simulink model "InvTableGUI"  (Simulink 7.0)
settings: Solver=FixedStepDiscrete  StartTime=0.0  StopTime=inf  FixedStep=samplePeriod  RelTol=1e-3
PreLoadFcn:
  | initialize
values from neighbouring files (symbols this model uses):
  forceCanon = 0.00444822    [initialize.m]    (also in TableInit.m = 1)
  iactParams = [	actParams    [initialize.m]
  inertia = inertia + inertiaP2Q([0 0 0], massA(i), cgA(:,i)-cg,  									inertiaCanon, massCanon)    [initialize.m]    (also in TableInit.m = [Ixx 0 0; 0 Iyy 0; 0 0 Izz])
  inertiaMask = zeros(3, 1)    [initialize.m]
  initDispl = zeros(6, 1)    [initialize.m]
  lengthCanon = 25.4    [initialize.m]    (also in TableInit.m)
  mass = ones(3, 1) * (sum(massA) + massT + massS)    [initialize.m]    (also in TableInit.m = 17300)
  massMask = zeros(3, 1)    [initialize.m]
  pitch = drot(2) * canon    [animation.m]    (also in positT2A.m = tbl(5))
  returnPress = 50    [initialize.m]    (also in TableInit.m)
  roll = drot(1) * canon    [animation.m]    (also in positT2A.m = tbl(4))
  rtg = cg    [initialize.m]    (also in TableInit.m = [0 0 cg])
  samplePeriod = controlPeriod/upsampleFactor    (= 0.00048828125)    [initialize.m]    (also in viewer.m = eval(getHeaderValue(header, 'DELTA_T')); TableInit.m = 0.0009765625)
  staticForce = forceT2A(ftbl, dtbl0, dof, rh, rb, rl, canon, atype)    [initialize.m]
undefined symbols (not defined in the file or in its folder): animation, atype, DiscIntNeverNeededParam, friction, yieldDispl
libraries: LibTransforms x15, LibDynamics x12, simulink x1

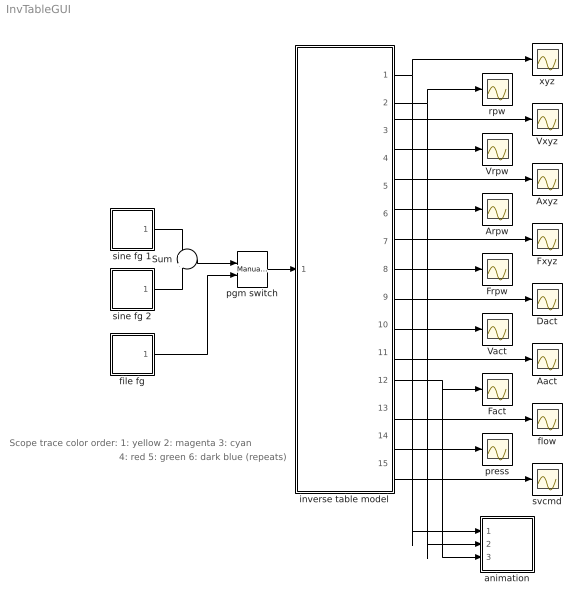
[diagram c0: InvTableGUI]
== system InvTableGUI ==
  note: Scope trace color order: 1: yellow 2: magenta 3: cyan
  note: 4: red 5: green 6: dark blue (repeats)
  Aact : Scope
  Arpw : Scope
  Axyz : Scope
  Dact : Scope
  Fact : Scope
  Frpw : Scope
  Fxyz : Scope
  Sum : Sum  Inputs=+|+  OutDataType=sfix(16)  OutScaling=2^0
  Vact : Scope
  Vrpw : Scope
  Vxyz : Scope
  animation : Subsystem  mask{azim=-37.5, elev=35, params=animation, decim=ceil((1/samplePeriod)/32), samplePeriod=samplePeriod}
      mask prompts: azim "View azimuth (degrees)"; elev "View elevation (degrees)"; params "Parameters"; decim "Decimation factor"; samplePeriod "Sample period (sec)"
  file fg : Subsystem
  flow : Scope
  inverse table model : Subsystem
  pgm switch : simulink/Signal Routing/Manual Switch  SystemSampleTime=-1  sw=1  action=0  varsize=off
  press : Scope
  rpw : Scope
  sine fg 1 : Subsystem  mask(Sine Function Generator){id=roll, ampl=500, freq=1, phase=0, spanInterval=1, samplePeriod=samplePeriod}
      mask prompts: id "DOF"; ampl "Amplitude"; freq "Frequency (Hz)"; phase "Phase (deg)"; spanInterval "Span interval (sec)"; samplePeriod "Sample period (sec)"
  sine fg 2 : Subsystem  mask(Sine Function Generator){id=pitch, ampl=500*0, freq=1, phase=90, spanInterval=1, samplePeriod=samplePeriod}
      mask prompts: id "DOF"; ampl "Amplitude"; freq "Frequency (Hz)"; phase "Phase (deg)"; spanInterval "Span interval (sec)"; samplePeriod "Sample period (sec)"
  svcmd : Scope
  xyz : Scope
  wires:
  pgm switch/1 -> inverse table model/1(Adof)
  inverse table model/1(xyz) -> xyz/1, animation/1(xyz)
  inverse table model/2(rpw) -> rpw/1, animation/2(rpw)
  file fg/1(out) -> pgm switch/2
  inverse table model/3(Vxyz) -> Vxyz/1
  inverse table model/4(Vrpw) -> Vrpw/1
  inverse table model/7(Fxyz) -> Fxyz/1
  inverse table model/8(Frpw) -> Frpw/1
  inverse table model/9(Dact) -> Dact/1
  inverse table model/10(Vact) -> Vact/1
  inverse table model/11(Aact) -> Aact/1
  inverse table model/12(Fact) -> Fact/1, animation/3(Fact)
  inverse table model/13(flow) -> flow/1
  inverse table model/14(press) -> press/1
  inverse table model/15(svcmd) -> svcmd/1
  inverse table model/6(Arpw) -> Arpw/1
  inverse table model/5(Axyz) -> Axyz/1
  Sum/1 -> pgm switch/1
  sine fg 1/1(out) -> Sum/1
  sine fg 2/1(out) -> Sum/2

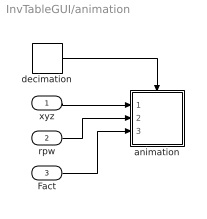
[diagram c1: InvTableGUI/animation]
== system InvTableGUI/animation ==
  xyz : Inport
  rpw : Inport  Port=2
  Fact : Inport  Port=3
  animation : Subsystem  TreatAsAtomicUnit=on
  decimation : DiscretePulseGenerator  Period=decim  SampleTime=samplePeriod
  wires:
  rpw/1 -> animation/2(rpw)
  Fact/1 -> animation/3(Fact)
  xyz/1 -> animation/1(xyz)
  decimation/1 -> animation/Trigger

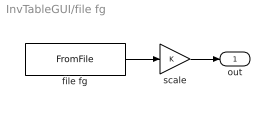
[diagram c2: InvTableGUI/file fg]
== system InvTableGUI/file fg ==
  file fg : FromFile  FileName=KobeAccel.mat  SampleTime=samplePeriod
  scale : Gain  ParameterDataType=sfix(16)  ParameterScaling=2^0  OutDataType=sfix(16)  OutScaling=2^0
  out : Outport  OutDataType=sfix(16)  OutScaling=2^0
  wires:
  scale/1 -> out/1
  file fg/1 -> scale/1

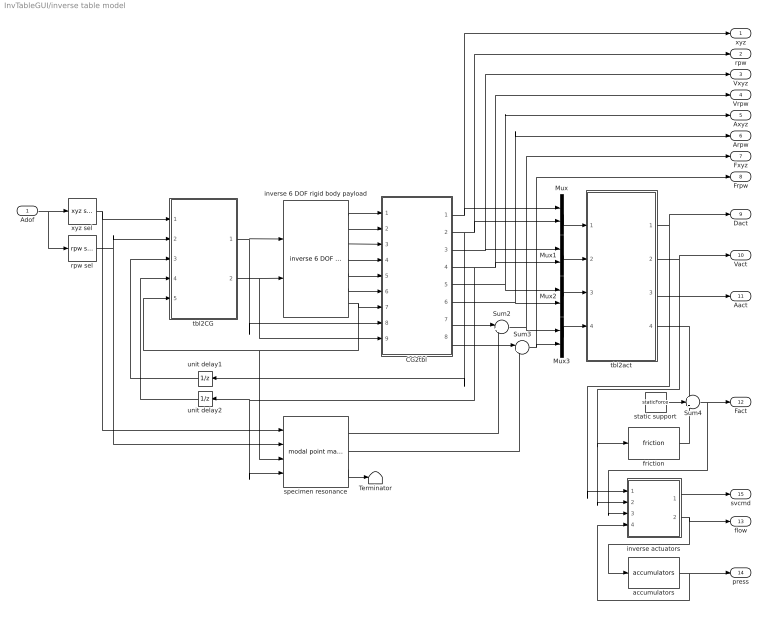
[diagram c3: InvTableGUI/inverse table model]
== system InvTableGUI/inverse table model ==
  Adof : Inport  PortDimensions=6  OutDataType=sfix(16)  OutScaling=2^0
  CG2tbl : Subsystem  mask{ofst=-rtg}
      mask prompts: ofst "Origin offset"
  Mux{,1..3} (4 alike) : Mux  Inputs=2
  Sum2 : Sum  Inputs=|++  OutDataType=sfix(16)  OutScaling=2^0
  Sum3 : Sum  Inputs=|++  OutDataType=sfix(16)  OutScaling=2^0
  Sum4 : Sum  Inputs=+-+  OutDataType=sfix(16)  OutScaling=2^0
  Terminator : Terminator
  accumulators : LibDynamics/accumulators  SystemSampleTime=-1  pumpFlow=pumpFlow  supplyPressure=supplyPress  precharge=precharge  bottleVolume=volume  gasConstant=gasConstant  flowCanon=flowCanon  volumeCanon=volumeCanon  samplePeriod=samplePeriod
  friction : LibDynamics/friction  SystemSampleTime=-1  friction=friction * forceCanon  yieldDispl=yieldDispl * lengthCanon  hysteresis=0  velocCanon=linVelocCanon  samplePeriod=samplePeriod
  inverse 6 DOF rigid body payload : LibDynamics/inverse 6 DOF rigid body payload  SystemSampleTime=-1  mass=mass.*massMask  inertia=diag(inertia.*inertiaMask)  gee=gee  massCanon=massCanon  inertiaCanon=inertiaCanon  linVelocCanon=linVelocCanon  linAccelCanon=linAccelCanon  rotDisplCanon=rotDisplCanon  rotVelocCanon=rotVelocCanon  rotAccelCanon=rotAccelCanon  rotForceCanon=rotForceCanon  initialPosition=initDispl  samplePeriod=samplePeriod
  inverse actuators : Subsystem
  rpw sel : LibTransforms/rpw sel  SystemSampleTime=-1  dof=1:6
  specimen resonance : LibDynamics/modal point mass  SystemSampleTime=-1  mass=modalMass  freq=modalFreq  damp=modalDamp  ofst=modalCG  gee=gee  massCanon=massCanon  linAccelCanon=linAccelCanon  rotDisplCanon=rotDisplCanon  rotVelocCanon=rotVelocCanon  rotForceCanon=rotForceCanon  samplePeriod=samplePeriod
  static support : Constant  Value=staticForce  OutDataType=sfix(16)  OutScaling=2^0
  tbl2CG : Subsystem  mask{ofst=rtg}
      mask prompts: ofst "Origin offset"
  tbl2act : Subsystem
  unit delay1 : UnitDelay  Orientation=left  X0=initDispl(4:6)  SampleTime=-1
  unit delay2 : UnitDelay  Orientation=left  SampleTime=-1
  xyz sel : LibTransforms/xyz sel  SystemSampleTime=-1  dof=1:6
  xyz : Outport  OutDataType=sfix(16)  OutScaling=2^0
  rpw : Outport  Port=2  OutDataType=sfix(16)  OutScaling=2^0
  Vxyz : Outport  Port=3  OutDataType=sfix(16)  OutScaling=2^0
  Vrpw : Outport  Port=4  OutDataType=sfix(16)  OutScaling=2^0
  Axyz : Outport  Port=5  OutDataType=sfix(16)  OutScaling=2^0
  Arpw : Outport  Port=6  OutDataType=sfix(16)  OutScaling=2^0
  Fxyz : Outport  Port=7  OutDataType=sfix(16)  OutScaling=2^0
  Frpw : Outport  Port=8  OutDataType=sfix(16)  OutScaling=2^0
  Dact : Outport  Port=9  OutDataType=sfix(16)  OutScaling=2^0
  Vact : Outport  Port=10  OutDataType=sfix(16)  OutScaling=2^0
  Aact : Outport  Port=11  OutDataType=sfix(16)  OutScaling=2^0
  Fact : Outport  Port=12  OutDataType=sfix(16)  OutScaling=2^0
  flow : Outport  Port=13  OutDataType=sfix(16)  OutScaling=2^0
  press : Outport  Port=14  OutDataType=sfix(16)  OutScaling=2^0
  svcmd : Outport  Port=15  OutDataType=sfix(16)  OutScaling=2^0
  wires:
  specimen resonance/2 -> Sum3/2
  specimen resonance/1 -> Sum2/2
  Sum3/1 -> Frpw/1, Mux3/2
  CG2tbl/8(Frpw) -> Sum3/1
  CG2tbl/7(Fxyz) -> Sum2/1
  Sum2/1 -> Fxyz/1, Mux3/1
  unit delay1/1 -> tbl2CG/3(rpw)
  unit delay2/1 -> tbl2CG/4(Vrpw)
  tbl2act/4(forceA) -> Sum4/1
  tbl2act/3(accelA) -> Aact/1
  tbl2act/2(velocA) -> Vact/1, inverse actuators/2(veloc), friction/1
  tbl2act/1(displA) -> Dact/1, inverse actuators/1(displ)
  Adof/1 -> rpw sel/1, xyz sel/1
  inverse 6 DOF rigid body payload/7 -> specimen resonance/3, tbl2CG/5(DCM), CG2tbl/7(DCM)
  inverse 6 DOF rigid body payload/6 -> CG2tbl/6(force rpw)
  inverse 6 DOF rigid body payload/5 -> CG2tbl/5(force xyz)
  inverse 6 DOF rigid body payload/4 -> CG2tbl/4(veloc rpw)
  inverse 6 DOF rigid body payload/3 -> CG2tbl/3(veloc xyz)
  inverse 6 DOF rigid body payload/2 -> CG2tbl/2(displ rpw)
  inverse 6 DOF rigid body payload/1 -> CG2tbl/1(displ xyz)
  Mux3/1 -> tbl2act/4(forceT)
  Mux2/1 -> tbl2act/3(accelT)
  Mux1/1 -> tbl2act/2(velocT)
  Mux/1 -> tbl2act/1(displT)
  CG2tbl/6(Arpw) -> Arpw/1, Mux2/2
  CG2tbl/5(Axyz) -> Axyz/1, Mux2/1
  CG2tbl/4(Vrpw) -> specimen resonance/4, unit delay2/1, Vrpw/1, Mux1/2
  CG2tbl/3(Vxyz) -> Vxyz/1, Mux1/1
  CG2tbl/2(rpw) -> unit delay1/1, rpw/1, Mux/2
  CG2tbl/1(xyz) -> xyz/1, Mux/1
  tbl2CG/2(accel rpw) -> CG2tbl/9(accel rpw), inverse 6 DOF rigid body payload/2
  rpw sel/1 -> specimen resonance/2, tbl2CG/2(Arpw)
  tbl2CG/1(accel xyz) -> CG2tbl/8(accel xyz), inverse 6 DOF rigid body payload/1
  inverse actuators/1(cmd) -> svcmd/1
  accumulators/1 -> press/1, inverse actuators/4(press)
  xyz sel/1 -> specimen resonance/1, tbl2CG/1(Axyz)
  inverse actuators/2(flow) -> flow/1, accumulators/1
  Sum4/1 -> Fact/1, inverse actuators/3(force)
  friction/1 -> Sum4/3
  static support/1 -> Sum4/2
  specimen resonance/3 -> Terminator/1

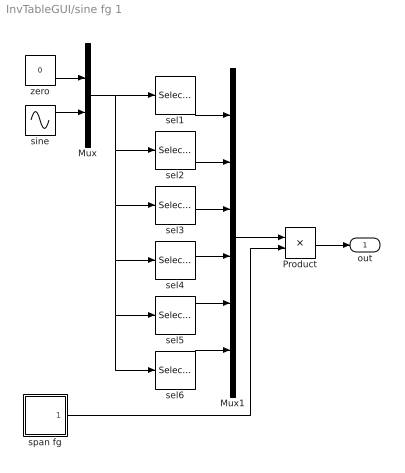
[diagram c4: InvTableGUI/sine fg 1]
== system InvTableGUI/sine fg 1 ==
  Mux : Mux  Inputs=2
  Mux1 : Mux  Inputs=6
  Product : Product  OutDataType=sfix(16)  OutScaling=2^0
  sel1 : Selector  InputPortWidth=2  IndexOptions=Index vector (dialog)  Indices=(id==1)+1  OutputSizes=1
  sel2 : Selector  InputPortWidth=2  IndexOptions=Index vector (dialog)  Indices=(id==2)+1  OutputSizes=1
  sel3 : Selector  InputPortWidth=2  IndexOptions=Index vector (dialog)  Indices=(id==3)+1  OutputSizes=1
  sel4 : Selector  InputPortWidth=2  IndexOptions=Index vector (dialog)  Indices=(id==4)+1  OutputSizes=1
  sel5 : Selector  InputPortWidth=2  IndexOptions=Index vector (dialog)  Indices=(id==5)+1  OutputSizes=1
  sel6 : Selector  InputPortWidth=2  IndexOptions=Index vector (dialog)  Indices=(id==6)+1  OutputSizes=1
  sine : Sin  Amplitude=ampl  Frequency=2 * pi * freq  Phase=phase*180/pi  SampleTime=samplePeriod
  span fg : Subsystem  mask{spanInterval=spanInterval, samplePeriod=samplePeriod}
      mask prompts: spanInterval "Span interval (sec)"; samplePeriod "Sample period (sec)"
  zero : Constant  Value=0  OutDataType=sfix(16)  OutScaling=2^0  SampleTime=samplePeriod
  out : Outport  OutDataType=sfix(16)  OutScaling=2^0
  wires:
  span fg/1(out) -> Product/2
  Product/1 -> out/1
  Mux1/1 -> Product/1
  zero/1 -> Mux/1
  sine/1 -> Mux/2
  sel1/1 -> Mux1/1
  sel2/1 -> Mux1/2
  sel3/1 -> Mux1/3
  sel4/1 -> Mux1/4
  sel5/1 -> Mux1/5
  sel6/1 -> Mux1/6
  Mux/1 -> sel2/1, sel3/1, sel4/1, sel5/1, sel6/1, sel1/1

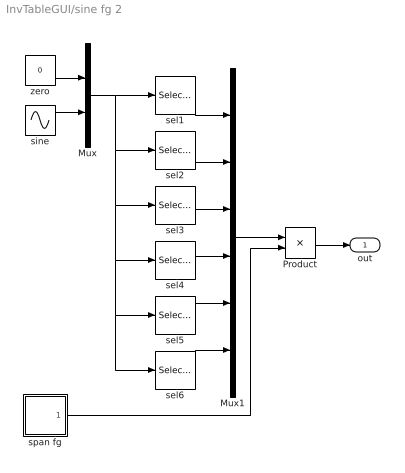
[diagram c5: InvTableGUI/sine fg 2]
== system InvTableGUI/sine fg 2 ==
  Mux : Mux  Inputs=2
  Mux1 : Mux  Inputs=6
  Product : Product  OutDataType=sfix(16)  OutScaling=2^0
  sel1 : Selector  InputPortWidth=2  IndexOptions=Index vector (dialog)  Indices=(id==1)+1  OutputSizes=1
  sel2 : Selector  InputPortWidth=2  IndexOptions=Index vector (dialog)  Indices=(id==2)+1  OutputSizes=1
  sel3 : Selector  InputPortWidth=2  IndexOptions=Index vector (dialog)  Indices=(id==3)+1  OutputSizes=1
  sel4 : Selector  InputPortWidth=2  IndexOptions=Index vector (dialog)  Indices=(id==4)+1  OutputSizes=1
  sel5 : Selector  InputPortWidth=2  IndexOptions=Index vector (dialog)  Indices=(id==5)+1  OutputSizes=1
  sel6 : Selector  InputPortWidth=2  IndexOptions=Index vector (dialog)  Indices=(id==6)+1  OutputSizes=1
  sine : Sin  Amplitude=ampl  Frequency=2 * pi * freq  Phase=phase*180/pi  SampleTime=samplePeriod
  span fg : Subsystem  mask{spanInterval=spanInterval, samplePeriod=samplePeriod}
      mask prompts: spanInterval "Span interval (sec)"; samplePeriod "Sample period (sec)"
  zero : Constant  Value=0  OutDataType=sfix(16)  OutScaling=2^0  SampleTime=samplePeriod
  out : Outport  OutDataType=sfix(16)  OutScaling=2^0
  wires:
  span fg/1(out) -> Product/2
  Product/1 -> out/1
  Mux1/1 -> Product/1
  zero/1 -> Mux/1
  sine/1 -> Mux/2
  sel1/1 -> Mux1/1
  sel2/1 -> Mux1/2
  sel3/1 -> Mux1/3
  sel4/1 -> Mux1/4
  sel5/1 -> Mux1/5
  sel6/1 -> Mux1/6
  Mux/1 -> sel2/1, sel3/1, sel4/1, sel5/1, sel6/1, sel1/1

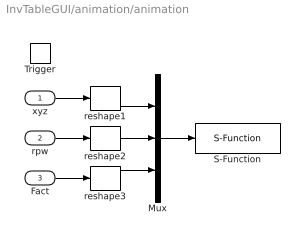
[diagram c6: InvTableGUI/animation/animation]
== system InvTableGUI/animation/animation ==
  xyz : Inport  OutDataType=sfix(16)  OutScaling=2^0
  rpw : Inport  Port=2  OutDataType=sfix(16)  OutScaling=2^0
  Fact : Inport  Port=3  OutDataType=sfix(16)  OutScaling=2^0
  Trigger : TriggerPort
  Mux : Mux  Inputs=3
  S-Function : S-Function  FunctionName=animation  Parameters=azim,elev,params
  reshape1 : Reshape
  reshape2 : Reshape
  reshape3 : Reshape
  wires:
  reshape1/1 -> Mux/1
  reshape2/1 -> Mux/2
  rpw/1 -> reshape2/1
  reshape3/1 -> Mux/3
  Fact/1 -> reshape3/1
  xyz/1 -> reshape1/1
  Mux/1 -> S-Function/1

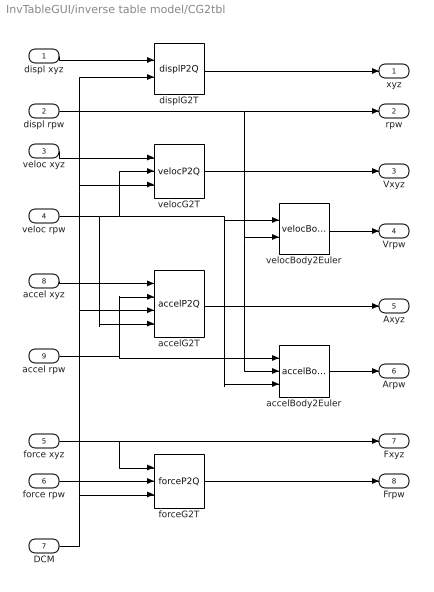
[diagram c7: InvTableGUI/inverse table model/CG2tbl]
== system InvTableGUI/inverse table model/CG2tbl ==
  displ xyz : Inport  OutDataType=sfix(16)  OutScaling=2^0
  displ rpw : Inport  Port=2  OutDataType=sfix(16)  OutScaling=2^0
  veloc xyz : Inport  Port=3  OutDataType=sfix(16)  OutScaling=2^0
  veloc rpw : Inport  Port=4  OutDataType=sfix(16)  OutScaling=2^0
  force xyz : Inport  Port=5  OutDataType=sfix(16)  OutScaling=2^0
  force rpw : Inport  Port=6  OutDataType=sfix(16)  OutScaling=2^0
  DCM : Inport  Port=7  OutDataType=sfix(16)  OutScaling=2^0
  accel xyz : Inport  Port=8  OutDataType=sfix(16)  OutScaling=2^0
  accel rpw : Inport  Port=9  OutDataType=sfix(16)  OutScaling=2^0
  accelBody2Euler : LibTransforms/accelBody2Euler  SystemSampleTime=-1  dof=1:6
  accelG2T : LibTransforms/accelP2Q  SystemSampleTime=-1  dof=1:6  ofst=ofst
  displG2T : LibTransforms/displP2Q  SystemSampleTime=-1  dof=1:6  ofst=ofst
  forceG2T : LibTransforms/forceP2Q  SystemSampleTime=-1  dof=1:6  ofst=ofst
  velocBody2Euler : LibTransforms/velocBody2Euler  SystemSampleTime=-1  dof=1:6
  velocG2T : LibTransforms/velocP2Q  SystemSampleTime=-1  dof=1:6  ofst=ofst
  xyz : Outport  OutDataType=sfix(16)  OutScaling=2^0
  rpw : Outport  Port=2  OutDataType=sfix(16)  OutScaling=2^0
  Vxyz : Outport  Port=3  OutDataType=sfix(16)  OutScaling=2^0
  Vrpw : Outport  Port=4  OutDataType=sfix(16)  OutScaling=2^0
  Axyz : Outport  Port=5  OutDataType=sfix(16)  OutScaling=2^0
  Arpw : Outport  Port=6  OutDataType=sfix(16)  OutScaling=2^0
  Fxyz : Outport  Port=7  OutDataType=sfix(16)  OutScaling=2^0
  Frpw : Outport  Port=8  OutDataType=sfix(16)  OutScaling=2^0
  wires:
  DCM/1 -> forceG2T/3, accelG2T/3, velocG2T/3, displG2T/2
  forceG2T/1 -> Frpw/1
  accelBody2Euler/1 -> Arpw/1
  accel rpw/1 -> accelG2T/2, accelBody2Euler/1
  accelG2T/1 -> Axyz/1
  accel xyz/1 -> accelG2T/1
  force rpw/1 -> forceG2T/2
  force xyz/1 -> Fxyz/1, forceG2T/1
  velocG2T/1 -> Vxyz/1
  veloc rpw/1 -> accelG2T/4, accelBody2Euler/3, velocBody2Euler/1, velocG2T/2
  velocBody2Euler/1 -> Vrpw/1
  veloc xyz/1 -> velocG2T/1
  displ rpw/1 -> velocBody2Euler/2, accelBody2Euler/2, rpw/1
  displG2T/1 -> xyz/1
  displ xyz/1 -> displG2T/1

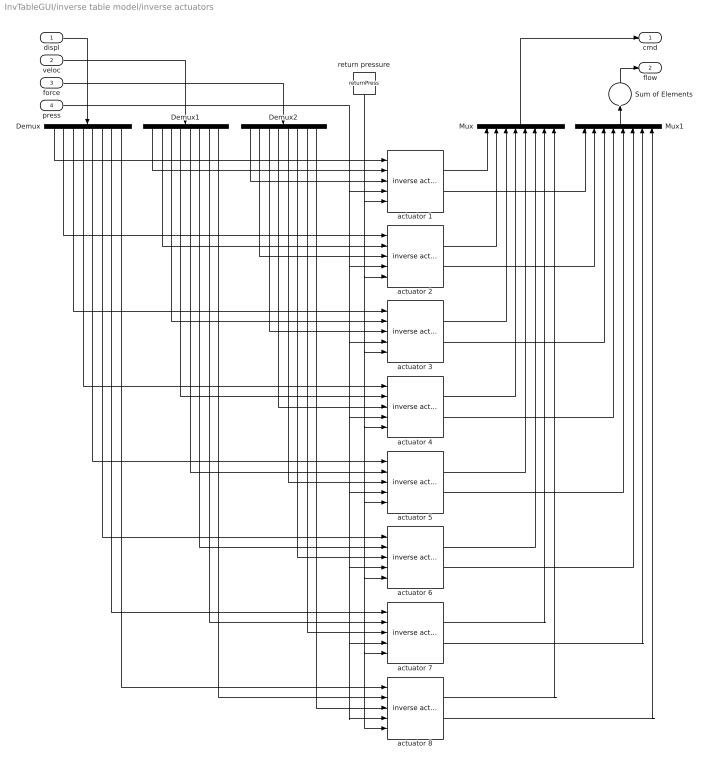
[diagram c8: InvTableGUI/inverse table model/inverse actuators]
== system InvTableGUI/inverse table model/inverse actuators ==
  displ : Inport  OutDataType=sfix(16)  OutScaling=2^0
  veloc : Inport  Port=2  OutDataType=sfix(16)  OutScaling=2^0
  force : Inport  Port=3  OutDataType=sfix(16)  OutScaling=2^0
  press : Inport  Port=4  OutDataType=sfix(16)  OutScaling=2^0
  Demux : Demux  Orientation=down  Outputs=nAct
  Demux1 : Demux  Orientation=down  Outputs=nAct
  Demux2 : Demux  Orientation=down  Outputs=nAct
  Mux : Mux  Orientation=up  Inputs=nAct
  Mux1 : Mux  Orientation=up  Inputs=nAct
  Sum of Elements : Sum  Orientation=up  Inputs=+  OutDataType=sfix(16)  OutScaling=2^-10
  actuator 1 : LibDynamics/inverse actuator  SystemSampleTime=-1  params=iactParams(:,1)
  actuator 2 : LibDynamics/inverse actuator  SystemSampleTime=-1  params=iactParams(:,2)
  actuator 3 : LibDynamics/inverse actuator  SystemSampleTime=-1  params=iactParams(:,3)
  actuator 4 : LibDynamics/inverse actuator  SystemSampleTime=-1  params=iactParams(:,4)
  actuator 5 : LibDynamics/inverse actuator  SystemSampleTime=-1  params=iactParams(:,5)
  actuator 6 : LibDynamics/inverse actuator  SystemSampleTime=-1  params=iactParams(:,6)
  actuator 7 : LibDynamics/inverse actuator  SystemSampleTime=-1  params=iactParams(:,7)
  actuator 8 : LibDynamics/inverse actuator  SystemSampleTime=-1  params=iactParams(:,8)
  return pressure : Constant  Orientation=down  Value=returnPress  OutDataType=sfix(16)  OutScaling=2^0
  cmd : Outport  OutDataType=sfix(16)  OutScaling=2^0
  flow : Outport  Port=2  OutDataType=sfix(16)  OutScaling=2^0
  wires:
  displ/1 -> Demux/1
  veloc/1 -> Demux1/1
  Demux/1 -> actuator 1/1
  Demux/2 -> actuator 2/1
  Demux1/1 -> actuator 1/2
  Demux2/1 -> actuator 1/3
  Demux1/2 -> actuator 2/2
  Demux2/2 -> actuator 2/3
  Demux/3 -> actuator 3/1
  Demux1/3 -> actuator 3/2
  Demux2/3 -> actuator 3/3
  Demux/4 -> actuator 4/1
  Demux1/4 -> actuator 4/2
  Demux2/4 -> actuator 4/3
  Demux/5 -> actuator 5/1
  Demux1/5 -> actuator 5/2
  Demux2/5 -> actuator 5/3
  Demux/6 -> actuator 6/1
  Demux1/6 -> actuator 6/2
  Demux2/6 -> actuator 6/3
  Demux/7 -> actuator 7/1
  Demux1/7 -> actuator 7/2
  Demux2/7 -> actuator 7/3
  Demux/8 -> actuator 8/1
  Demux1/8 -> actuator 8/2
  Demux2/8 -> actuator 8/3
  actuator 3/1 -> Mux/3
  actuator 4/1 -> Mux/4
  actuator 5/1 -> Mux/5
  actuator 6/1 -> Mux/6
  actuator 7/1 -> Mux/7
  actuator 8/1 -> Mux/8
  actuator 1/1 -> Mux/1
  actuator 2/1 -> Mux/2
  actuator 1/2 -> Mux1/1
  actuator 2/2 -> Mux1/2
  actuator 3/2 -> Mux1/3
  actuator 4/2 -> Mux1/4
  actuator 5/2 -> Mux1/5
  actuator 6/2 -> Mux1/6
  actuator 7/2 -> Mux1/7
  actuator 8/2 -> Mux1/8
  Mux1/1 -> Sum of Elements/1
  press/1 -> actuator 7/4, actuator 8/4, actuator 6/4, actuator 5/4, actuator 4/4, actuator 3/4, actuator 2/4, actuator 1/4
  return pressure/1 -> actuator 7/5, actuator 8/5, actuator 6/5, actuator 5/5, actuator 4/5, actuator 3/5, actuator 2/5, actuator 1/5
  Sum of Elements/1 -> flow/1
  Mux/1 -> cmd/1
  force/1 -> Demux2/1

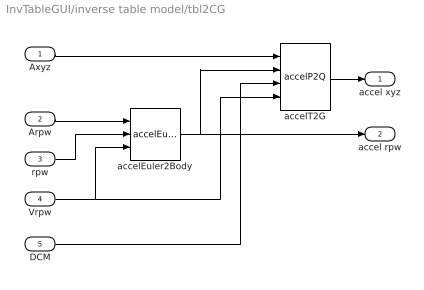
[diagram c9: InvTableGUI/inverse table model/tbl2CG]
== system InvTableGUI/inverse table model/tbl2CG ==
  Axyz : Inport  OutDataType=sfix(16)  OutScaling=2^0
  Arpw : Inport  Port=2  OutDataType=sfix(16)  OutScaling=2^0
  rpw : Inport  Port=3  OutDataType=sfix(16)  OutScaling=2^0
  Vrpw : Inport  Port=4  OutDataType=sfix(16)  OutScaling=2^0
  DCM : Inport  Port=5  OutDataType=sfix(16)  OutScaling=2^0
  accelEuler2Body : LibTransforms/accelEuler2Body  SystemSampleTime=-1  dof=1:6
  accelT2G : LibTransforms/accelP2Q  SystemSampleTime=-1  dof=1:6  ofst=ofst
  accel xyz : Outport  OutDataType=sfix(16)  OutScaling=2^0
  accel rpw : Outport  Port=2  OutDataType=sfix(16)  OutScaling=2^0
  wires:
  DCM/1 -> accelT2G/3
  rpw/1 -> accelEuler2Body/2
  Vrpw/1 -> accelEuler2Body/3, accelT2G/4
  accelEuler2Body/1 -> accel rpw/1, accelT2G/2
  Arpw/1 -> accelEuler2Body/1
  accelT2G/1 -> accel xyz/1
  Axyz/1 -> accelT2G/1

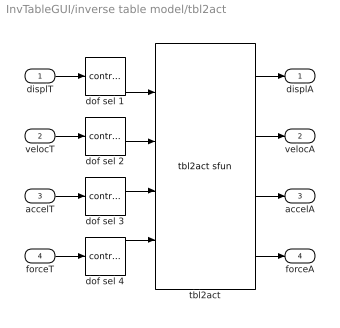
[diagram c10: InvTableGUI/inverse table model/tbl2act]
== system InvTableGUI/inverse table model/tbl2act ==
  displT : Inport
  velocT : Inport  Port=2
  accelT : Inport  Port=3
  forceT : Inport  Port=4
  dof sel {1..4} (4 alike) : LibTransforms/contract  SystemSampleTime=-1  elements=dof
  tbl2act : LibTransforms/tbl2act sfun  atype=atype  nVel=length(atype)  nFrc=length(atype)  dof=dof  rh=rh  rb=rb  rl=rl  ra=ra  ea=ea  offset=[0 0 0 0 0 0]  fmax=fmax  canon=canon  gee=gee  action=1  rate=0
  displA : Outport
  velocA : Outport  Port=2
  accelA : Outport  Port=3
  forceA : Outport  Port=4
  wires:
  displT/1 -> dof sel 1/1
  tbl2act/1 -> displA/1
  velocT/1 -> dof sel 2/1
  tbl2act/2 -> velocA/1
  accelT/1 -> dof sel 3/1
  tbl2act/3 -> accelA/1
  forceT/1 -> dof sel 4/1
  tbl2act/4 -> forceA/1
  dof sel 1/1 -> tbl2act/1
  dof sel 2/1 -> tbl2act/2
  dof sel 3/1 -> tbl2act/3
  dof sel 4/1 -> tbl2act/4

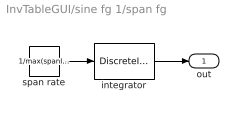
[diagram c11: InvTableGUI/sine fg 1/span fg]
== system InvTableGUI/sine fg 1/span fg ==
  integrator : DiscreteIntegrator  SampleTime=samplePeriod  OutDataType=sfix(16)  OutScaling=2^0  LimitOutput=on  UpperSaturationLimit=1  LowerSaturationLimit=0  ICPrevOutput=DiscIntNeverNeededParam  ICPrevScaledInput=DiscIntNeverNeededParam
  span rate : Constant  Value=1/max(spanInterval,samplePeriod)  OutDataType=sfix(16)  OutScaling=2^0  SampleTime=samplePeriod
  out : Outport  OutDataType=sfix(16)  OutScaling=2^0
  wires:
  span rate/1 -> integrator/1
  integrator/1 -> out/1

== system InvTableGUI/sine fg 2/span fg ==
  integrator : DiscreteIntegrator  SampleTime=samplePeriod  OutDataType=sfix(16)  OutScaling=2^0  LimitOutput=on  UpperSaturationLimit=1  LowerSaturationLimit=0  ICPrevOutput=DiscIntNeverNeededParam  ICPrevScaledInput=DiscIntNeverNeededParam
  span rate : Constant  Value=1/max(spanInterval,samplePeriod)  OutDataType=sfix(16)  OutScaling=2^0  SampleTime=samplePeriod
  out : Outport  OutDataType=sfix(16)  OutScaling=2^0
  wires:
  span rate/1 -> integrator/1
  integrator/1 -> out/1
